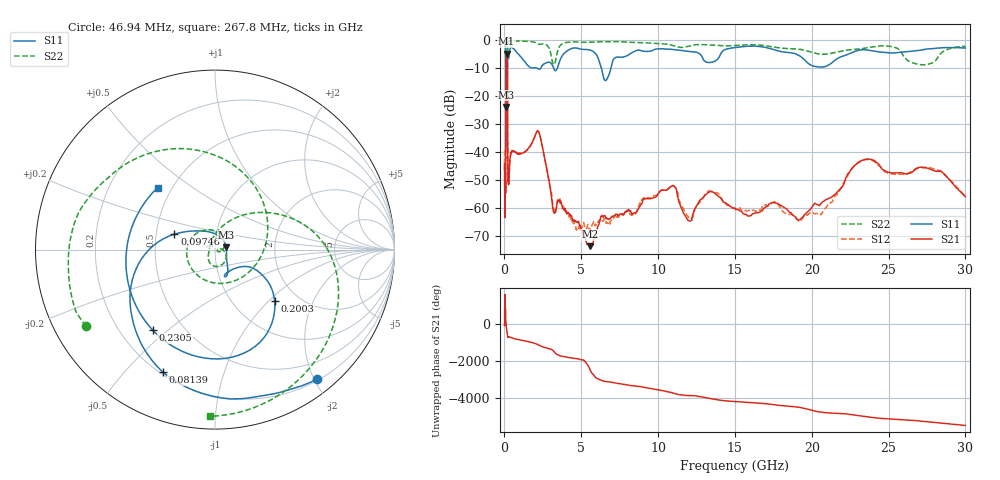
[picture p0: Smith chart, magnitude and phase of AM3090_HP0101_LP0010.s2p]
! Date/Time: Thu, Feb 28, 2019 1:58 PM
! Network Analyzer: Agilent Technologies E8364B Rev: A.07.50.67
! Sweep from 0.010 to 30.000 GHz, 1601 Points, Sweep Type: LOG
! Power Supply: 5.023 V, 0.002 A
# Hz S DB R 50
!freq MagS11 AngS11 MagS21 AngS21 MagS12 AngS12 MagS22 AngS22
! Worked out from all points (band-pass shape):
!   1601 points, 10 MHz to 30 GHz, reference 50 ohm
!   highest |S21| = -4.85 dB at 141.8 MHz (marker M1); lowest = -73.6 dB at 5.556 GHz (marker M2)
!   |S21| within 3 dB of the highest: 106.3 MHz to 184.7 MHz (78.4 MHz wide, 53.9 % of centre)
!   lowest |S11| = -23.9 dB at 105.1 MHz (marker M3), VSWR 1.14, Z = 56.7 + j1.36 ohm
!   |S11| at or under -10 dB: 2.067 GHz to 2.361 GHz (294.4 MHz wide, 13.3 % of centre); 3.201 GHz to 3.448 GHz (246.8 MHz wide, 7.42 % of centre); 6.308 GHz to 6.932 GHz (624.5 MHz wide, 9.43 % of centre)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
!   |S22| runs from -38.1 to -0.2 dB; largest |S21 - S12| = 0.015
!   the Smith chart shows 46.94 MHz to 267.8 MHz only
!   S11 on the Smith chart (normalised r, x): 46.94 MHz: 0.23, -2.04; 81.39 MHz: 0.21, -0.64; 97.46 MHz: 0.62, +0.11; 200.3 MHz: 1.54, -1.08; 230.5 MHz: 0.34, -0.44; 267.8 MHz: 0.42, +0.37
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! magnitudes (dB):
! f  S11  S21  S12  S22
! 10 MHz  -0.2  -46.1  -39.5  -0.5
! 38.04 MHz  -0.5  -60.1  -58.7  -1.3
! 46.94 MHz  -0.8  -51.0  -50.2  -1.6
! 81.39 MHz  -2.6  -48.7  -47.4  -5.5
! 97.46 MHz  -12.3  -15.2  -15.2  -15.0
! 105.1 MHz  -23.9  -8.4  -8.4  -17.1
! 131.6 MHz  -16.2  -5.0  -5.0  -37.9
! 141.8 MHz  -16.7  -4.9  -4.8  -27.4
! 144.7 MHz  -16.8  -4.9  -4.8  -24.6
! 178.6 MHz  -14.5  -6.7  -6.6  -30.0
! 200.3 MHz  -7.2  -18.8  -18.8  -9.3
! 230.5 MHz  -4.9  -49.8  -49.6  -1.5
! 267.8 MHz  -6.6  -51.7  -51.4  -0.6
! 550.5 MHz  -3.0  -39.7  -39.8  -0.2
! 2.084 GHz  -10.0  -33.0  -33.0  -1.0
! 3.236 GHz  -10.5  -61.7  -60.7  -8.8
! 5.556 GHz  -3.5  -73.6  -67.6  -0.8
! 7.926 GHz  -5.7  -61.1  -61.3  -0.7
! 10.76 GHz  -3.3  -52.8  -52.6  -1.7
! 19.8 GHz  -8.5  -61.0  -62.1  -4.1
! 23.48 GHz  -3.5  -42.6  -42.8  -2.9
! 30 GHz  -2.9  -56.0  -55.8  -2.2
